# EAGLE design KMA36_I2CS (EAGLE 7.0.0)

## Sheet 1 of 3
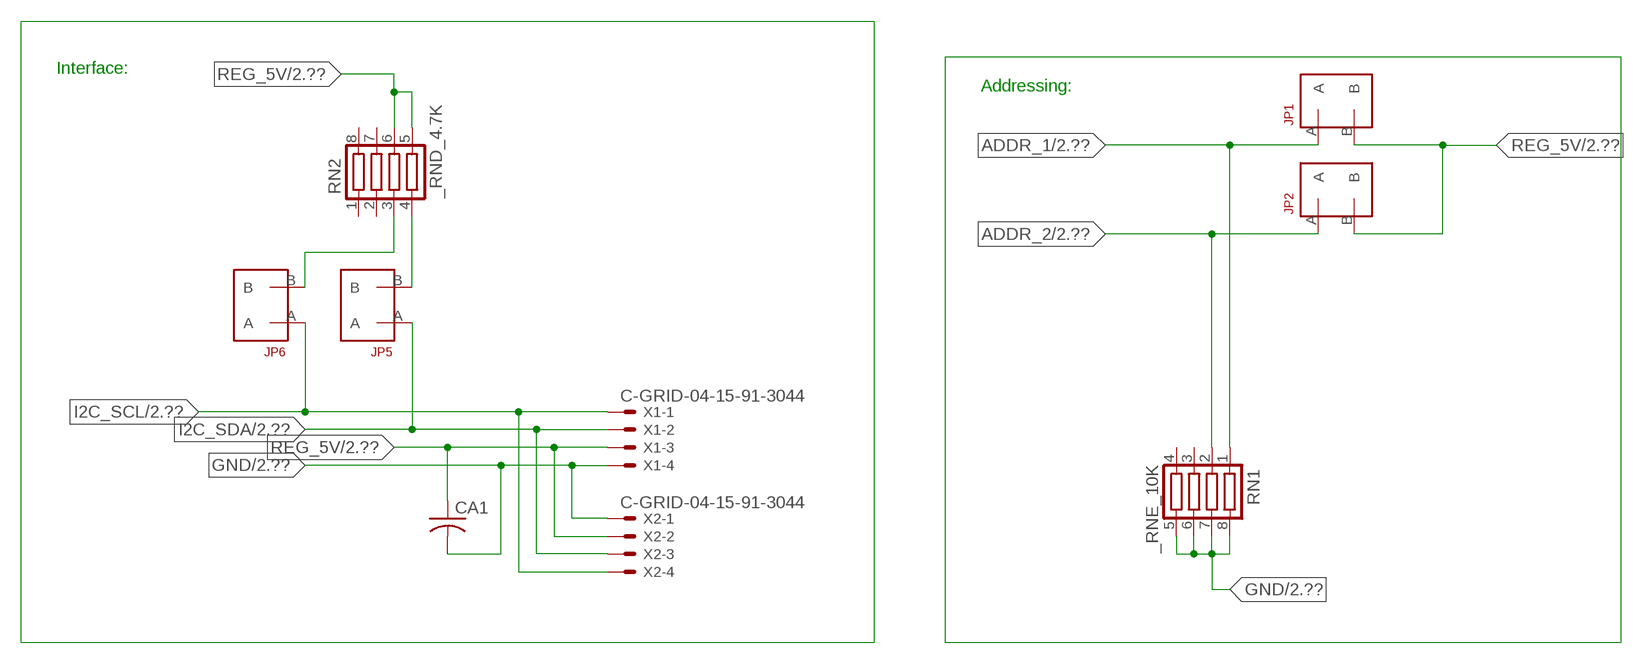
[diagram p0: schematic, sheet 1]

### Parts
CA1  CC1206KRX7R9BB104  [.1UF]
JP1  JUMPER_1X2_2MM  [JUMPER_1X2_2MM]
JP2  JUMPER_1X2_2MM  [JUMPER_1X2_2MM]
JP5  JUMPER_1X2_2MM  [JUMPER_1X2_2MM]
JP6  JUMPER_1X2_2MM  [JUMPER_1X2_2MM]
RN1  _RNE_10K  [RNE]
RN2  _RND_4.7K  [RND]
X1  C-GRID-04-15-91-3044  [15-91-04]
X2  C-GRID-04-15-91-3044  [15-91-04]

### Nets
ADDR_1: JP1.A RN1.1 ; also sheet 2
ADDR_2: JP2.A RN1.2 ; also sheet 2
GND: CA1.2 RN1.5 RN1.6 RN1.7 RN1.8 X1.4 X2.1 ; also sheet 2,3
I2C_SCL: JP6.A X1.1 X2.4 ; also sheet 2
I2C_SDA: JP5.A X1.2 X2.3 ; also sheet 2
N$1: JP6.B RN2.3
N$2: JP5.B RN2.4
REG_5V: CA1.1 JP1.B JP2.B RN2.5 RN2.6 X1.3 X2.2 ; also sheet 2,3
Unconnected: RN1.3 RN1.4 RN2.1 RN2.2 RN2.7 RN2.8

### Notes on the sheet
- Interface:
- Addressing:

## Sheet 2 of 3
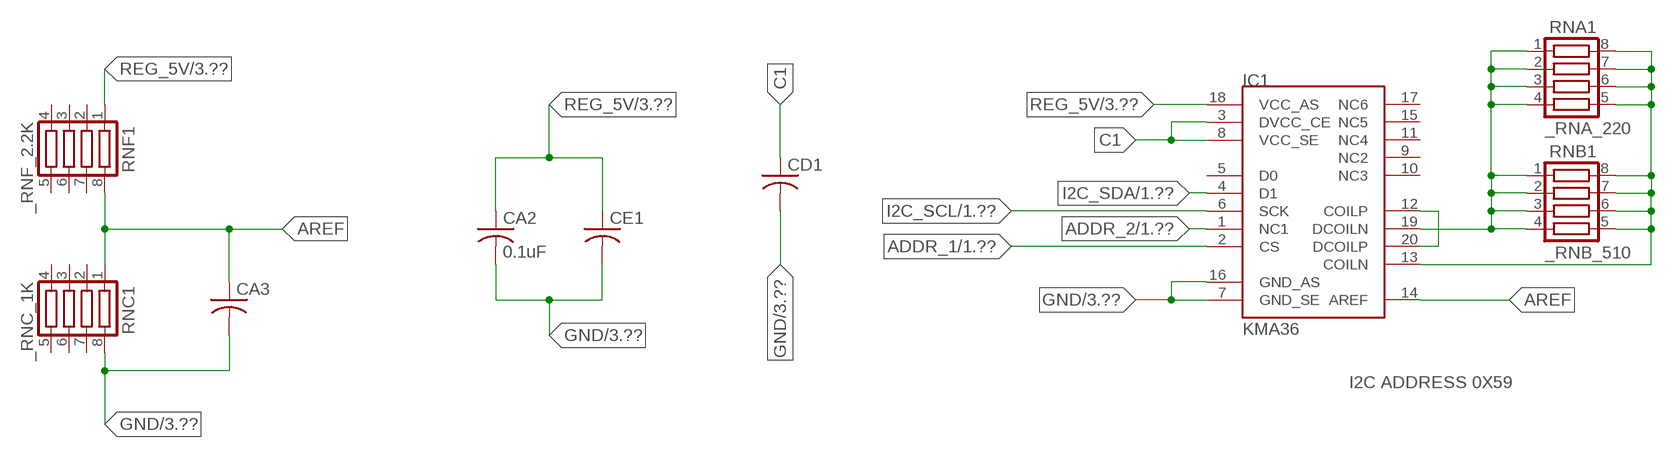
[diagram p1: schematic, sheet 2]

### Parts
CA2  0.1uF  CC1206KRX7R9BB104C1206K  [CC1206KRX7R9BB104]
CA3  CC1206KRX7R9BB104  [.1UF]
CD1  CC1206KRX7R9BB103C1206K  [CC1206KRX7R9BB103]
CE1  CC0603JRNPO8BN1020603  [CC0603JRNPO8BN102]
IC1  KMA36  [KMA36]
RNA1  _RNA_220  [RNA]
RNB1  _RNB_510  [RNB]
RNC1  _RNC_1K  [RNC]
RNF1  _RNF_2.2K  [RNF]

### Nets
ADDR_1: IC1.2(CS) ; also sheet 1
ADDR_2: IC1.1(NC1) ; also sheet 1
AREF: CA3.1 IC1.14(AREF) RNC1.1 RNF1.8
C1: CD1.1 IC1.3(DVCC_CE) IC1.8(VCC_SE)
GND: CA2.2 CA3.2 CD1.2 CE1.2 IC1.7(GND_SE) IC1.16(GND_AS) RNC1.8 ; also sheet 1,3
I2C_SCL: IC1.6(SCK) ; also sheet 1
I2C_SDA: IC1.4(D1) ; also sheet 1
N$5: IC1.12(COILP) IC1.20(DCOILP)
N$7: IC1.19(DCOILN) RNA1.1 RNA1.2 RNA1.3 RNA1.4 RNB1.1 RNB1.2 RNB1.3 RNB1.4
N$8: IC1.13(COILN) RNA1.5 RNA1.6 RNA1.7 RNA1.8 RNB1.5 RNB1.6 RNB1.7 RNB1.8
REG_5V: CA2.1 CE1.1 IC1.18(VCC_AS) RNF1.1 ; also sheet 1,3
Unconnected: IC1.5(D0) IC1.9(NC2) IC1.10(NC3) IC1.11(NC4) IC1.15(NC5) IC1.17(NC6) RNC1.2 RNC1.3 RNC1.4 RNC1.5 RNC1.6 RNC1.7 RNF1.2 RNF1.3 RNF1.4 RNF1.5 RNF1.6 RNF1.7

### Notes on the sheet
- I2C ADDRESS 0X59

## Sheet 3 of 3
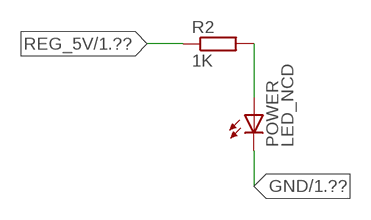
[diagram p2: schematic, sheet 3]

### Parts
POWER  LED_NCD  [CHIPLED_0603]
R2  1K  RESISTOR_SMT-0402  [R402]

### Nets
GND: POWER.C ; also sheet 1,2
N$3: POWER.A R2.2
REG_5V: R2.1 ; also sheet 1,2

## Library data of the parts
CA1-CA3 = NCD_ULTIMATE_LIBRARY:CC1206KRX7R9BB104: Capacitor CA .1uF 50V SMT C1206K CC1206KRX7R9BB104
CD1 = NCD_ULTIMATE_LIBRARY:CC1206KRX7R9BB103: Capacitor CD .01uF SMT CC1206KRX7R9BB103 1206
CE1 = NCD_ULTIMATE_LIBRARY:CC0603JRNPO8BN102: Capacitor CE 1uF SMT CC0603JRNPO8BN102 0603
IC1 = NCD_ULTIMATE_AMAN:KMA36
JP1 JP2 JP5 JP6 = NCD_ULTIMATE_CONNECTORS:JUMPER_1X2_2MM
POWER = NCD_ULTIMATE_LIBRARY:LED_NCD: LED Digikey 754-1132-2-ND/APT2012SRCPRV
R2 = NCD_ULTIMATE_LIBRARY:RESISTOR_SMT: NCD Resistor
RN1 = NCD_ULTIMATE_LIBRARY:_RNE_10K: Resistor Array RNE SMT 10K x 4 Single Resistor Source: http://www.ctscorp.com/components/Datasheets/CTSChipArrayDs.pdf Digikey 742C083103JPTR-ND/742C083103JP; OC_FARNELL: unknown; OC_NEWARK: unknown
RN2 = NCD_ULTIMATE_LIBRARY:_RND_4.7K: Resistor Array RND SMT 4.7K x 4 Single Resistor Source: http://www.ctscorp.com/components/Datasheets/CTSChipArrayDs.pdf Digikey 742C083472JPTR-ND/742C083472JP; OC_FARNELL: unknown; OC_NEWARK: unknown
RNA1 = NCD_ULTIMATE_LIBRARY:_RNA_220: Resistor Array RNA SMT 220 x 4 Single Resistor Source: http://www.ctscorp.com/components/Datasheets/CTSChipArrayDs.pdf Digikey 742C083221JPTR-ND/742C083221JP; OC_FARNELL: unknown; OC_NEWARK: unknown
RNB1 = NCD_ULTIMATE_LIBRARY:_RNB_510: Resistor Array RNB SMT 510 x 4 Single Resistor Source: http://www.ctscorp.com/components/Datasheets/CTSChipArrayDs.pdf Digikey 742C083511JPTR-ND/ 742C083511JP; OC_FARNELL: unknown; OC_NEWARK: unknown
RNC1 = NCD_ULTIMATE_LIBRARY:_RNC_1K: Resistor Array RNC SMT 1K x 4 Single Resistor Source: http://www.ctscorp.com/components/Datasheets/CTSChipArrayDs.pdf Digikey 742C083102JPTR-ND/742C083102JP; OC_FARNELL: unknown; OC_NEWARK: unknown
RNF1 = NCD_ULTIMATE_LIBRARY:_RNF_2.2K: Resistor Array RNF SMT 2.2K x 4 Single Resistor Source: http://www.ctscorp.com/components/Datasheets/CTSChipArrayDs.pdf Digikey 742C083222JPTR-ND/742C083222JP; OC_FARNELL: unknown; OC_NEWARK: unknown
X1 X2 = NCD_ULTIMATE_CONNECTORS:C-GRID-04: CONNECTOR 4-Pos I2C wire to board 2.54 mm (0.100") pitch header Digikey WM1342-ND/0015912045; OC_FARNELL: unknown; OC_NEWARK: unknown

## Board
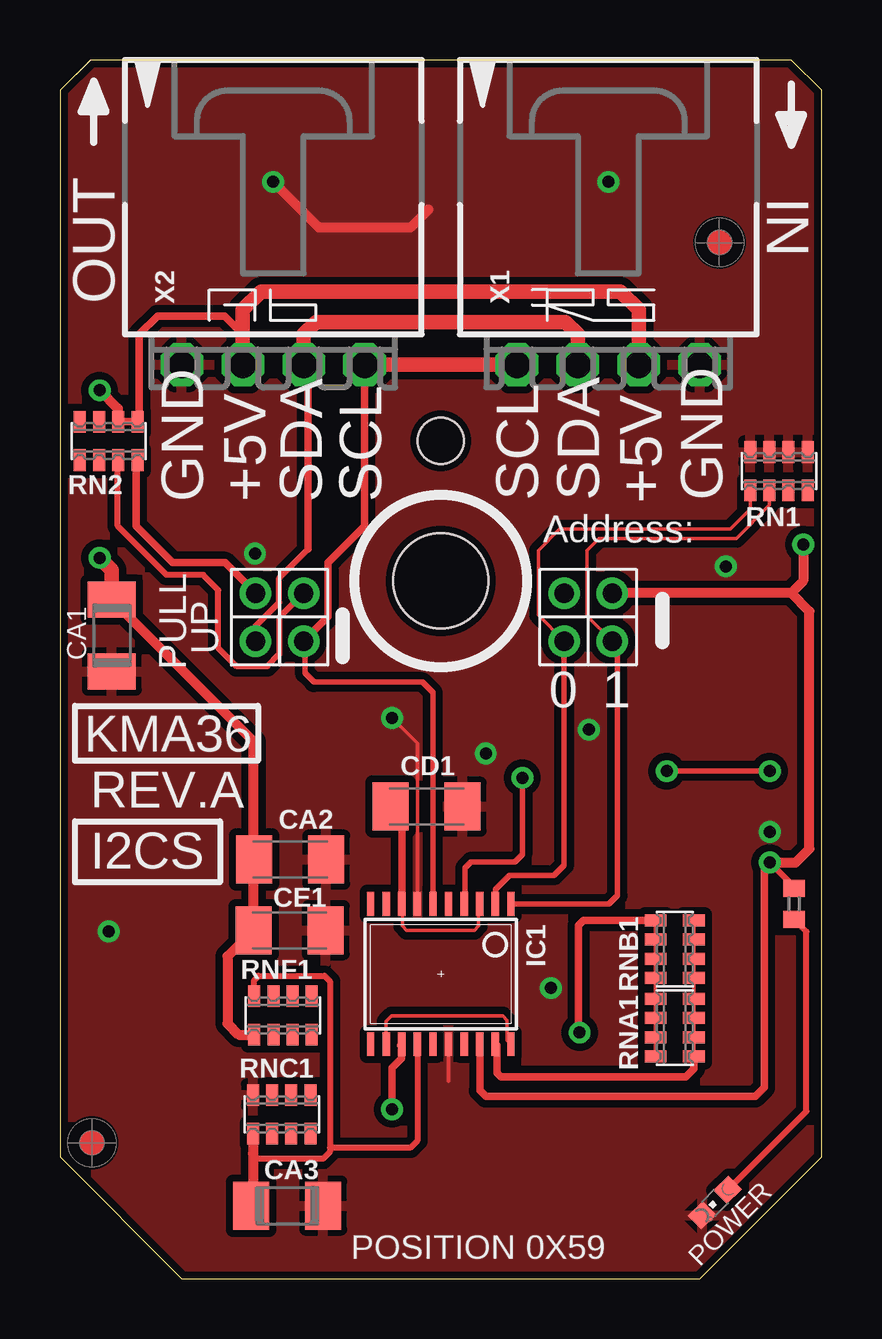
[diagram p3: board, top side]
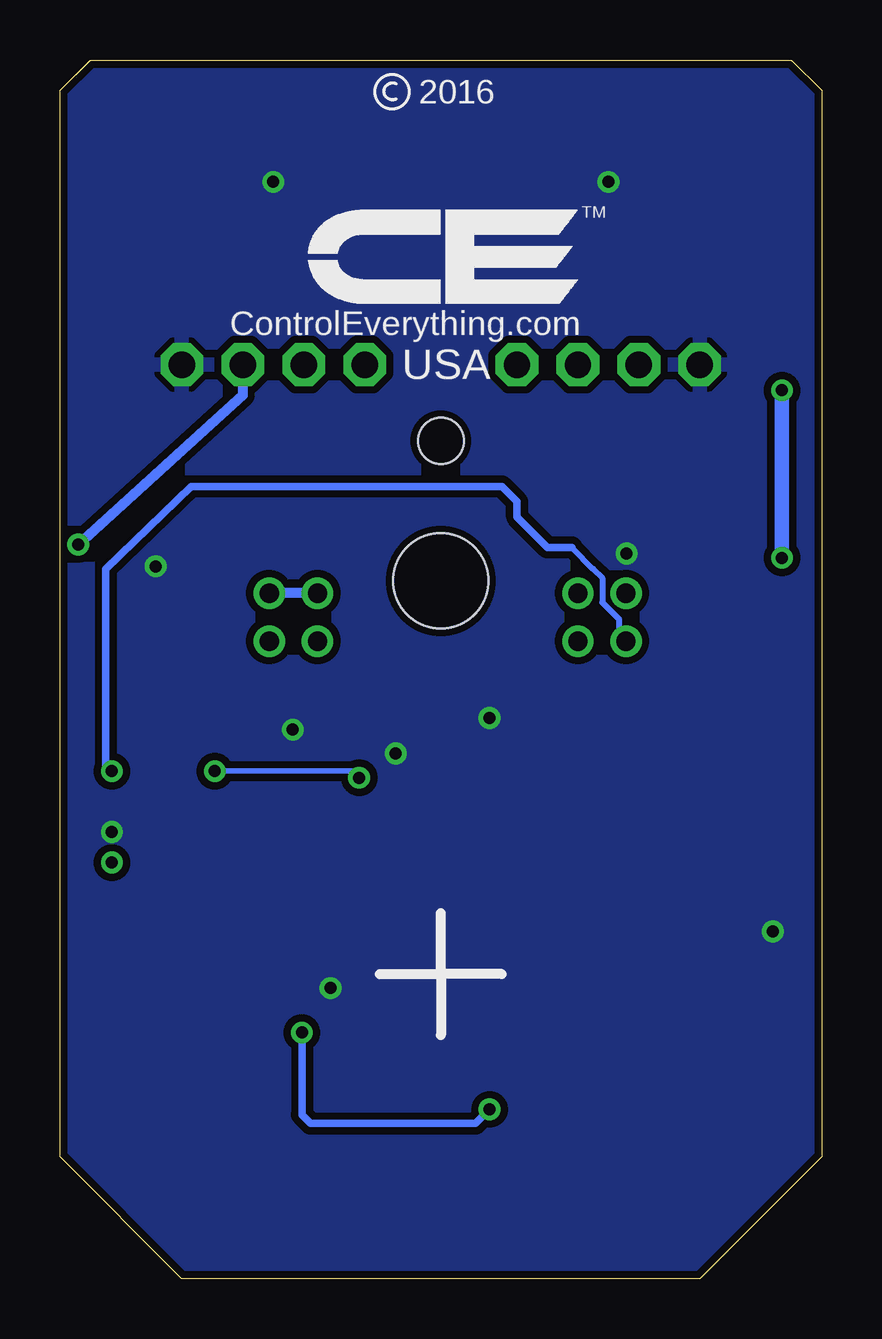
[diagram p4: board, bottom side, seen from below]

Size 31.75 x 50.8 mm. Coordinates in mm from the lower left corner, seen from the top.
Outline: 31.75,5.08 31.75,49.53 30.48,50.8 1.27,50.8 0,49.53 0,5.08 5.08,0 26.67,0 31.75,5.08
Outline: 31.75,5.08 31.75,49.53 30.48,50.8 1.27,50.8 0,49.53 0,5.08 5.08,0 26.67,0 31.75,5.08
Copper layers (1*16): Top 0.035mm / dielectric 1.5mm / Bottom 0.035mm
Design rules "default": minimum track width 5mil, minimum drill 24mil, track to track 5mil, track to pad 5mil, pad to pad 5mil, via to via 5mil, smd to smd 5mil, copper to edge 10mil, drill to drill 8mil, minimum pad ring 10mil, minimum via ring 8mil, stop-mask expansion 2mil, vias tented up to drill 0mil, thermal gap 10mil
Holes 3.96 mm at 15.88,29.08
Holes 1.91 mm at 15.88,34.92

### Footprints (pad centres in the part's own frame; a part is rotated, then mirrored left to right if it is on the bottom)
.1UF = smd 1.5 x 2: 1 -1.5,0; 2 1.5,0
CC1206KRX7R9BB104 = smd 1.5 x 2: 1 -1.5,0; 2 1.5,0
CC1206KRX7R9BB103 = smd 1.5 x 2: 1 -1.5,0; 2 1.5,0
CC0603JRNPO8BN102 = smd 1.5 x 2: 1 -1.5,0; 2 1.5,0
KMA36 = smd 0.305 x 0.991: 1 -2.925,-2.918; 2 -2.275,-2.918; 3 -1.625,-2.918; 4 -0.975,-2.918; 5 -0.325,-2.918; 6 0.325,-2.918; 7 0.975,-2.918; 8 1.625,-2.918; 9 2.275,-2.918; 10 2.925,-2.918; 11 2.925,2.918; 12 2.275,2.918; 13 1.625,2.918; 14 0.975,2.918; 15 0.325,2.918; 16 -0.325,2.918; 17 -0.975,2.918; 18 -1.625,2.918; 19 -2.275,2.918; 20 -2.925,2.918
JUMPER_1X2_2MM = drill 0.8: A 0,2; B 0,0
CHIPLED_0603 = smd 0.8 x 0.876: A 0,-0.75; C 0,0.75
R402 = smd 0.7 x 0.9: 1 -0.65,0; 2 0.65,0
RNE = smd 0.5 x 0.9: 1 -1.2,-0.8; 2 -0.4,-0.8; 3 0.4,-0.8; 4 1.2,-0.8; 5 1.2,0.8; 6 0.4,0.8; 7 -0.4,0.8; 8 -1.2,0.8
RND = smd 0.5 x 0.9: 1 -1.2,-0.8; 2 -0.4,-0.8; 3 0.4,-0.8; 4 1.2,-0.8; 5 1.2,0.8; 6 0.4,0.8; 7 -0.4,0.8; 8 -1.2,0.8
RNA = smd 0.5 x 0.9: 1 -1.2,-0.8; 2 -0.4,-0.8; 3 0.4,-0.8; 4 1.2,-0.8; 5 1.2,0.8; 6 0.4,0.8; 7 -0.4,0.8; 8 -1.2,0.8
RNB = smd 0.5 x 0.9: 1 -1.2,-0.8; 2 -0.4,-0.8; 3 0.4,-0.8; 4 1.2,-0.8; 5 1.2,0.8; 6 0.4,0.8; 7 -0.4,0.8; 8 -1.2,0.8
RNC = smd 0.5 x 0.9: 1 -1.2,-0.8; 2 -0.4,-0.8; 3 0.4,-0.8; 4 1.2,-0.8; 5 1.2,0.8; 6 0.4,0.8; 7 -0.4,0.8; 8 -1.2,0.8
RNF = smd 0.5 x 0.9: 1 -1.2,-0.8; 2 -0.4,-0.8; 3 0.4,-0.8; 4 1.2,-0.8; 5 1.2,0.8; 6 0.4,0.8; 7 -0.4,0.8; 8 -1.2,0.8
15-91-04 = drill 1.1 pad 1.778 octagon: 1 -3.81,-7.62; 2 -1.27,-7.62; 3 1.27,-7.62; 4 3.81,-7.62

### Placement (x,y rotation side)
CA1  2.16,26.81 270 top
CA2  9.6,17.48 0 top
CA3  9.47,3.05 0 top
CD1  15.29,19.69 0 top
CE1  9.58,14.53 0 top
IC1  15.88,12.7 180 top
JP1  21.02,28.58 180 top
JP2  23.03,28.58 180 top
JP5  8.15,28.58 180 top
JP6  10.16,28.58 180 top
POWER  27.3,3.18 135 top
R2  30.61,15.62 270 top
RN1  29.97,33.66 0 top
RN2  2.03,34.92 0 top
RNA1  25.63,10.46 90 top
RNB1  25.63,13.74 90 top
RNC1  9.25,6.86 0 top
RNF1  9.3,10.97 0 top
U$5  [VISION_REF10]  1.33,5.66 90 top
U$28  [VISION_REF10]  27.5,43.19 90 top
X1  22.86,45.72 0 top
X2  8.89,45.72 0 top

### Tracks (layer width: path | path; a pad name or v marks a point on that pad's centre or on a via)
ADDR_1
  Top 0.152: RN1.1 28.77,32.07 27.94,31.24 20.83,31.24 19.94,30.35 19.94,27.65 JP1.A
  Top 0.229: JP1.A 21.02,17.23 20.6,16.82 18.74,16.82 18.15,16.22 IC1.2
ADDR_2
  Top 0.152: RN1.2 29.57,32.24 28.19,30.86 22.48,30.86 21.97,30.35 21.97,27.63 JP2.A
  Top 0.229: IC1.1 22.88,15.62 23.24,15.98 23.24,26.36 JP2.A
AREF
  Top 0.254: RNF1.8 8.1,12.44 8.28,12.62 11.02,12.62 11.25,12.4 11.25,5.46 | 11.25,5.46 11.25,5.28 10.97,5 8.25,5 8.05,5.21 | IC1.14 14.9,5.76 14.6,5.46 11.25,5.46
  Top 0.406: RNC1.1 8.05,5.21 8.05,3.12 CA3.1
C1
  Top 0.152: IC1.3 17.45,15.57 17.45,14.71 17.27,14.53 14.45,14.53 14.27,14.71 14.27,15.59 IC1.8
  Top 0.305: IC1.8 14.25,19.23 CD1.1
GND  (via drill 0.5)
  Top 0.152: IC1.7 14.9,22.31 v13.84,23.37 | IC1.16 16.2,8.24 16.21,8.23
  Top 0.406: 15.35,44.57 14.6,43.82 10.8,43.82 v8.89,45.72
  other vias: 22.86,45.72 29.59,18.62 2.03,14.48 8.13,30.23 22.05,22.89 17.75,21.89 27.76,29.69 20.47,12.12
  pour Top (isolate 0.305): -1.27,0 -1.27,50.8 33.02,50.8 33.02,0
  pour Bottom (isolate 0.305): -5.08,0 -5.08,50.8 35.56,50.8 35.56,0
I2C_SCL
  Top 0.229: JP6.A 10.21,26.52 10.21,25.25 10.59,24.87 15.11,24.87 15.55,24.43 IC1.6
  Top 0.305: JP6.A 11.18,27.61 11.18,29.85 12.7,31.37 X2.4
  Top 0.406: X2.4 12.57,38.1 | 18.92,38.1 X1.1
  Top 0.61: 12.57,38.1 18.92,38.1
I2C_SDA  (via drill 0.5)
  Top 0.229: v29.59,21.16 v25.3,21.16 | v25.3,21.16 | v19.28,20.88 19.28,17.68 18.97,17.37 17.15,17.37 16.89,17.12 16.89,15.66 IC1.4
  Top 0.254: JP5.A 8.15,27.2 9.14,28.19 9.14,29.21 10.35,30.42
  Top 0.305: 10.35,30.42 10.35,37.91 X2.3
  Top 0.61: X2.3 10.16,39.37 10.67,39.88 21.08,39.88 21.59,39.37 X1.2
  Bottom 0.229: v25.3,21.16 19.56,21.16 v19.28,20.88
  Bottom 0.254: 10.41,30.48 9.52,29.59 9.14,29.21 9.14,28.19 8.45,27.5 8.45,26.87 JP5.A
  Bottom 0.305: 10.41,30.48 11.43,30.48 12.7,31.75 12.7,32.39 13.34,33.02 26.29,33.02 29.85,29.59 29.85,21.41 v29.59,21.16
N$1
  Top 0.254: JP6.B | JP6.B 9.14,27.56 9.14,26.04 8.64,25.53 7.37,25.53 6.6,26.29 6.6,28.7 5.97,29.34 4.45,29.34 2.41,31.37 2.41,34.11 RN2.3
N$2
  Top 0.305: JP5.B 6.88,29.85 4.7,29.85 3.18,31.37 3.18,34.07 RN2.4
N$3
  Top 0.254: POWER.A 31.12,6.99 31.12,14.46 R2.2
N$5
  Top 0.152: IC1.12 13.6,10.73 13.82,10.95 18.47,10.95 18.64,10.77 18.64,9.94 IC1.20
N$7
  Top 0.152: RNA1.1 RNA1.2 RNA1.3 RNA1.4 RNB1.1 RNB1.2 RNB1.3 RNB1.4
  Top 0.305: 18.16,9.77 IC1.19 18.21,9.72 18.21,8.59 18.39,8.41 26.09,8.41 26.43,8.75 RNA1.1
N$8  (via drill 0.5)
  Top 0.152: RNB1.5 RNB1.6 RNB1.7 RNB1.8 RNA1.5 RNA1.6 RNA1.7 RNA1.8
  Top 0.305: RNB1.5 21.83,14.94 21.62,14.73 21.62,10.31 v21.67,10.26 | 14.2,9.73 IC1.13 14.25,9.2 13.84,8.79 v13.84,7.06
  Bottom 0.305: v21.67,10.26 21.67,6.83 21.31,6.48 14.43,6.48 v13.84,7.06
REG_5V  (via drill 0.5)
  Top 0.254: v29.59,17.35 30.61,16.33 R2.1
  Top 0.305: 7.62,39.37 7.49,39.37 | RN2.6 RN2.5 3.3,35.8 3.3,39.37 4.06,40.13 6.86,40.13 7.62,39.37 | X2.2 7.62,39.37 | 2.16,28.09 CA1.1 | 29.54,17.3 v29.59,17.35 29.36,17.12 29.36,7.98 28.98,7.6 17.76,7.6 17.5,7.85 IC1.18 | JP2.B
  Top 0.406: v29.59,17.35 30.67,17.35 31.24,17.92 31.24,27.81 30.48,28.58 | v1.65,37.03 2.41,36.27 2.41,35.74 RN2.6 | v30.99,30.61 30.99,29.08 30.48,28.58 | 30.48,28.58 JP2.B | RNF1.1 7.46,10.17 6.99,10.64 6.99,13.44 CE1.1 8.08,17.45 | 8.08,17.45 8.08,22.39 CA1.1 | 8.08,17.45 CA2.1
  Top 0.61: X1.3 24.13,40.39 23.37,41.15 8.38,41.15 7.62,40.39 X2.2 | CA1.1 2.16,29.54 v1.65,30.05
  Bottom 0.406: v30.99,30.61 24.13,36.83 24.13,37.47 24.16,38.08 24.13,38.23 X1.3 | JP1.B JP2.B
  Bottom 0.61: v1.65,30.05 v1.65,37.03

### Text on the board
tNames: IN | OUT | GND | +5V | SDA | SCL | SCL | SDA | +5V | GND | Address: | UP | PULL | 0 | 1 | KMA36 | REV.A | I2CS | POSITION 0X59
bNames: 2016 | TM | ControlEverything.com | USA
